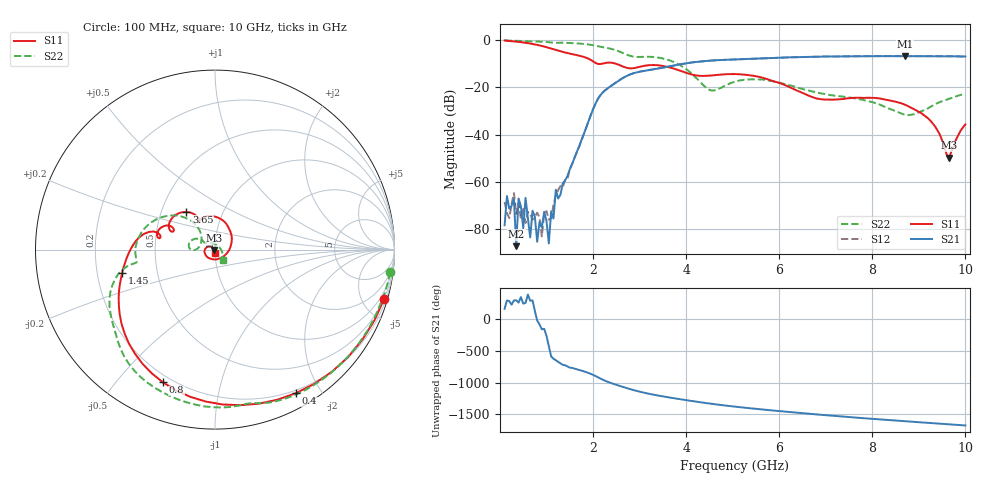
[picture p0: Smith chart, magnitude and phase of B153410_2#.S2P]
!  2-Port S-parameters saved by WinCal
! VAR MeasName=S-Parameters (CALIBRATED_DATA) read from VNA (N5245A)
! VAR MeasDate=2016-12-23 9:59:22
! VAR NAME=B153410_2#
! VAR FILENAME=B153410_2#.S2P
! VAR DATE=2016-12-23 9:59:22
! VAR PHYS_PORTS=1,2
# Hz S DB R 50
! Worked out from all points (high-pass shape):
!   199 points, 100 MHz to 10 GHz, reference 50 ohm
!   highest |S21| = -6.74 dB at 8.7 GHz (marker M1); lowest = -87.2 dB at 350 MHz (marker M2)
!   |S21| within 3 dB of the highest: 4.024 GHz to end of sweep
!   lowest |S11| = -49.7 dB at 9.65 GHz (marker M3), VSWR 1.01, Z = 49.7 - j0.138 ohm
!   |S11| at or under -10 dB: 2.096 GHz to 2.19 GHz (93.7 MHz wide, 4.37 % of centre); 2.49 GHz to end of sweep
!   |S22| runs from -31.8 to -0.1 dB; largest |S21 - S12| = 0.0023
!   S11 on the Smith chart (normalised r, x): 100 MHz: 0.46, -6.99; 400 MHz: 0.17, -1.70; 800 MHz: 0.17, -0.67; 1.45 GHz: 0.31, -0.11; 3.65 GHz: 0.67, +0.30; 10 GHz: 1.00, -0.03
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1e8  -0.16 -16.2  -78.37 152.4  -68.53 20.0  -0.13 -7.4
1.5e8  -0.25 -23.9  -65.97 -76.5  -73.04 108.7  -0.17 -10.9
3e8  -0.52 -46.3  -67.30 -77.8  -64.73 76.4  -0.28 -21.0
3.5e8  -0.63 -53.5  -87.21 -74.7  -73.63 52.4  -0.31 -24.3
4e8  -0.74 -60.5  -67.00 -110.1  -69.03 -59.8  -0.33 -27.6
5e8  -0.99 -74.1  -79.58 -126.6  -70.63 -92.9  -0.39 -34.2
5.5e8  -1.13 -80.7  -66.76 -114.9  -77.41 -102.7  -0.42 -37.5
6.5e8  -1.43 -93.5  -83.51 -81.8  -73.57 -49.2  -0.48 -44.1
7e8  -1.60 -99.7  -72.21 -75.5  -75.96 70.3  -0.52 -47.4
8e8  -2.00 -111.4  -85.34 -31.2  -73.03 -76.9  -0.59 -53.9
9e8  -2.46 -122.4  -79.32 -167.9  -83.09 -124.0  -0.68 -60.5
1.45e9  -5.47 -166.0  -57.53 -27.9  -58.91 -23.7  -1.15 -93.9
1.75e9  -6.82 176.6  -42.31 -93.3  -42.57 -94.4  -1.52 -113.5
2.25e9  -9.73 168.0  -21.37 110.4  -21.38 110.3  -3.11 -145.1
3.4e9  -10.65 139.3  -12.01 -124.0  -12.01 -124.1  -7.38 169.7
3.65e9  -11.57 127.3  -11.07 -155.2  -11.07 -155.3  -8.60 153.6
5.05e9  -14.36 103.9  -8.15 62.4  -8.18 62.4  -17.55 -179.7
6.7e9  -24.00 -30.5  -7.03 -52.7  -7.04 -52.6  -21.70 144.6
8.35e9  -25.40 174.4  -6.77 -147.1  -6.75 -147.0  -28.91 104.3
8.7e9  -27.33 158.8  -6.74 -165.5  -6.75 -165.6  -31.52 62.6
9.65e9  -49.74 -154.7  -6.82 146.0  -6.84 146.0  -24.79 -39.1
1e10  -35.63 -89.3  -6.93 128.5  -6.94 128.6  -22.67 -53.4
